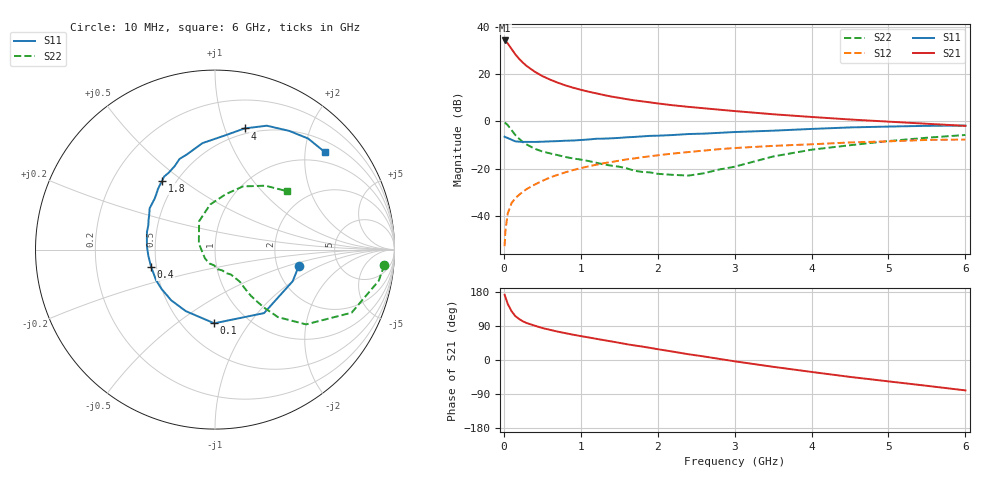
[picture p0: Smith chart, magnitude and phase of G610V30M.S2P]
! SIEMENS Small Signal Semiconductors
! BFG193
! Si NPN RF Bipolar Junction Transistor in SOT223
! VCE = 10 V  IC = 30 mA
! Common Emitter S-Parameters:  August  1996
# GHz  S  MA  R  50
!  f  S11  S21  S12  S22
! GHz  MAG  ANG  MAG  ANG  MAG  ANG  MAG  ANG
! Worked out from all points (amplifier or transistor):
!   36 points, 10 MHz to 6 GHz, reference 50 ohm
!   highest |S21| = 34.3 dB at 10 MHz (marker M1)
!   |S21| within 3 dB of that: start of sweep to 87.73 MHz
!   unconditionally stable (mu >= 1): 650.2 MHz to 2.495 GHz
!   at 250 MHz: K = 0.81, MSG = 27.2 dB, |S12| = -29.7 dB
!   at 1.4 GHz: K = 1.04, MAG = 12.5 dB, |S12| = -17.1 dB
!   at 6 GHz: K = 0.89, MSG = 2.9 dB, |S12| = -7.7 dB
!   S11 on the Smith chart (normalised r, x): 10 MHz: 2.65, -0.61; 100 MHz: 0.71, -0.70; 400 MHz: 0.47, -0.11; 1.8 GHz: 0.42, +0.42; 4 GHz: 0.45, +1.17; 6 GHz: 0.74, +2.44
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0.01  0.4761 -10.8  51.73 172.2  0.0023 87.9  0.9474 -5.2
0.02  0.4672 -22.2  50.53 166.3  0.0048 80.9  0.9284 -10.8
0.05  0.4471 -52.3  44.76 148.2  0.0112 72.4  0.8383 -24.8
0.1  0.4107 -90.6  34.31 129.0  0.0187 65.7  0.6563 -39.4
0.15  0.3795 -115.3  26.17 115.7  0.0238 62.0  0.5145 -47.0
0.2  0.3733 -130.7  21.06 108.0  0.0282 62.4  0.4286 -49.6
0.25  0.3698 -143.6  17.38 101.8  0.0329 62.2  0.3627 -51.3
0.3  0.3699 -152.6  14.79 97.3  0.0374 63.5  0.3238 -52.2
0.4  0.3687 -164.7  11.34 90.7  0.0461 64.3  0.2657 -52.5
0.5  0.373 -174.8  9.135 84.4  0.0553 63.8  0.2319 -52.2
0.6  0.3794 177.6  7.693 79.6  0.0653 63.6  0.2113 -53.1
0.7  0.3836 171.7  6.632 74.9  0.0742 62.9  0.194 -54.7
0.9  0.3953 160.0  5.185 66.8  0.0938 60.0  0.1652 -57.3
1.1  0.4152 152.0  4.271 59.6  0.112 57.3  0.1457 -64.6
1.4  0.44 139.8  3.36 48.9  0.1389 51.6  0.116 -76.1
1.8  0.4834 127.6  2.664 35.4  0.1752 43.5  0.0856 -98.3
2.2  0.5168 115.7  2.199 22.0  0.2094 34.5  0.0742 -138.6
3.5  0.6385 85.0  1.421 -17.9  0.3044 4.2  0.1816 119.1
4  0.6949 76.3  1.245 -31.5  0.329 -5.5  0.2526 96.1
4.5  0.7483 67.3  1.101 -44.6  0.3597 -15.5  0.3142 79.1
5.5  0.8076 50.0  0.894 -68.1  0.4067 -38.7  0.453 51.8
6  0.8185 41.5  0.807 -80.2  0.4143 -52.1  0.5176 38.9
